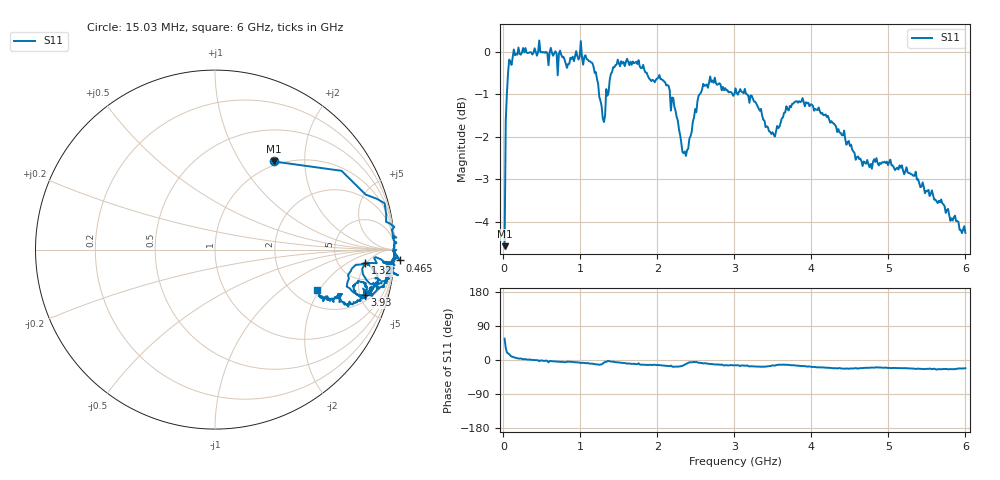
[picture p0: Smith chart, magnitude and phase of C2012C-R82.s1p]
!	Network	Analyzer	HP8753E.07.74:	Oct	30	2002	Serial	No.	JP38451487
!	Hewlett-Packard
!	28	Aug	2009	12:49:19
!	Frequency	S11
#	HZ	S	RI	R	50
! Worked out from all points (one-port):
!   400 points, 15.03 MHz to 6 GHz, reference 50 ohm
!   lowest |S11| = -4.6 dB at 15.03 MHz (marker M1), VSWR 3.88, Z = 47 + j70.9 ohm
!   |S11| at or under -10 dB: nowhere
!   S11 on the Smith chart (normalised r, x): 15.03 MHz: 0.94, +1.42; 465 MHz: -14, -27; 1.32 GHz: 9, -5; 3.93 GHz: 2.62, -5.55; 6 GHz: 2.64, -1.91
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1.502992e7  0.328 0.491
3.002985e7  0.705 0.439
4.502978e7  0.84 0.306
7.502962e7  0.945 0.258
1.650292e8  0.99 0.0912
4.650277e8  1.03 -0.0602
5.550272e8  1 -0.0224
5.850271e8  0.959 -0.104
6.750266e8  1 -0.0621
7.050265e8  0.936 -0.0714
7.650262e8  0.983 -0.0768
1.005025e9  1.02 -0.143
1.230024e9  0.897 -0.192
1.320023e9  0.838 -0.0734
1.395023e9  0.94 -0.0658
1.515022e9  0.955 -0.116
2.02502e9  0.914 -0.217
2.265019e9  0.792 -0.248
2.370018e9  0.741 -0.141
2.475018e9  0.834 -0.0727
2.685017e9  0.92 -0.171
3.015015e9  0.879 -0.22
3.525012e9  0.768 -0.205
3.765011e9  0.845 -0.204
3.93001e9  0.835 -0.253
4.515007e9  0.72 -0.294
5.265004e9  0.667 -0.271
6e9  0.569 -0.226
